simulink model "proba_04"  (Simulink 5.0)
settings: Solver=VariableStepDiscrete  SolverMode=SingleTasking  StartTime=0.0  StopTime=20.0  RelTol=1e-3  AbsTol=1e-6

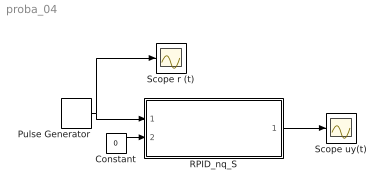
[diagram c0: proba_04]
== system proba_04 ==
  Constant : Constant  Value=0
  Pulse Generator : DiscretePulseGenerator  PulseType=Time based  Period=100  PulseWidth=50
  RPID_nq_S : Subsystem  mask( PID ){P=1, I=5, D=1, h=1}
      mask prompts: P "P :"; I "I [s]:"; D "D [s]:"; h "h [s]:"
      mask help: PID P, I, D - h - ;
      mask init:
      | %  Initialization commands
      |    t=@1;x=@2;u=@3;flag=@4;
      |    flag=0;
      | [sys,x0]=DPIDrc_S(t,x,u,flag,P,I,D,h);
  Scope r (t) : Scope
  Scope uy(t) : Scope
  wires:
  Pulse Generator/1 -> RPID_nq_S/1(In1), Scope r (t)/1
  Constant/1 -> RPID_nq_S/2(In2)
  RPID_nq_S/1(Out1) -> Scope uy(t)/1

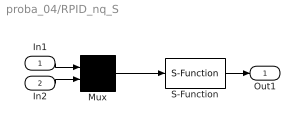
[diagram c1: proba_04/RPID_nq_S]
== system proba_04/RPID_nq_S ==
  In1 : Inport
  In2 : Inport  Port=2
  Mux : Mux  Inputs=2
  S-Function : S-Function  FunctionName=DPIDrc_S  Parameters=P,I,D,h
  Out1 : Outport  InitialOutput=0
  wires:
  Mux/1 -> S-Function/1
  In1/1 -> Mux/1
  S-Function/1 -> Out1/1
  In2/1 -> Mux/2
